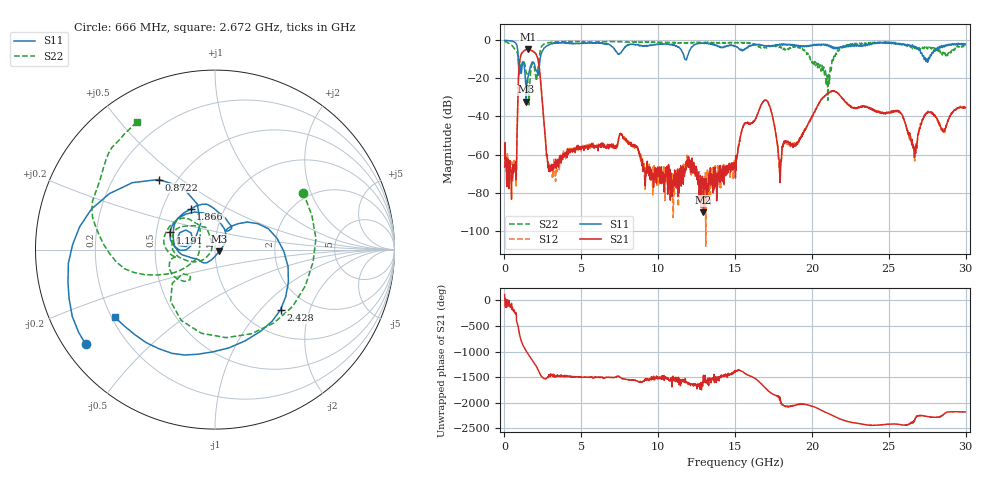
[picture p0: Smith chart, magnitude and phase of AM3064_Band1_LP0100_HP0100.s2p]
# Hz S DB R 50.0
!freq dBS11 angS11 dBS21 angS21 dBS12 angS12 dBS22 angS22
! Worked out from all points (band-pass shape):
!   1600 points, 10 MHz to 29.98 GHz, reference 50 ohm
!   highest |S21| = -4.62 dB at 1.528 GHz (marker M1); lowest = -90.3 dB at 12.94 GHz (marker M2)
!   |S21| within 3 dB of the highest: 1.075 GHz to 2.077 GHz (1.003 GHz wide, 63.6 % of centre)
!   lowest |S11| = -32.2 dB at 1.416 GHz (marker M3), VSWR 1.05, Z = 52.3 - j1.08 ohm
!   |S11| at or under -10 dB: 902.1 MHz to 2.314 GHz (1.412 GHz wide, 87.8 % of centre); 11.76 GHz to 11.84 GHz (80.56 MHz wide, 0.683 % of centre); 27.3928 GHz to 27.45994 GHz (67.14 MHz wide, 0.245 % of centre)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
!   |S22| runs from -33.9 to -0.4 dB; largest |S21 - S12| = 0.0091
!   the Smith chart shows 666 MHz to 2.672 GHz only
!   S11 on the Smith chart (normalised r, x): 666 MHz: 0.06, -0.33; 872.2 MHz: 0.40, +0.42; 1.191 GHz: 0.59, +0.12; 1.866 GHz: 0.69, +0.34; 2.428 GHz: 1.46, -1.30; 2.672 GHz: 0.21, -0.29
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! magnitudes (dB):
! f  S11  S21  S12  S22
! 10 MHz  -0.1  -66.6  -54.9  -0.4
! 666 MHz  -1.0  -66.0  -65.1  -4.6
! 872.2 MHz  -6.0  -30.9  -30.8  -8.4
! 1.191 GHz  -11.4  -6.2  -6.1  -10.8
! 1.416 GHz  -32.2  -4.8  -4.7  -16.8
! 1.528 GHz  -19.5  -4.6  -4.6  -22.1
! 1.866 GHz  -11.6  -5.8  -5.9  -12.1
! 2.428 GHz  -6.1  -29.0  -28.9  -3.0
! 2.672 GHz  -3.4  -53.4  -52.2  -1.6
! 3.028 GHz  -1.8  -67.1  -67.2  -1.0
! 5.015 GHz  -1.4  -56.2  -56.5  -0.7
! 7.639 GHz  -5.6  -49.9  -49.9  -0.7
! 10 GHz  -2.0  -68.6  -69.8  -1.0
! 12.94 GHz  -1.5  -90.3  -75.5  -1.1
! 15 GHz  -3.0  -66.0  -63.4  -1.4
! 16.9 GHz  -2.9  -31.5  -31.5  -3.8
! 17.93 GHz  -2.1  -74.8  -69.3  -3.1
! 19.99 GHz  -2.9  -40.4  -40.2  -11.1
! 25 GHz  -1.0  -37.8  -37.9  -1.2
! 26.68 GHz  -3.1  -59.6  -63.4  -4.2
! 27.45 GHz  -10.3  -38.2  -38.2  -3.6
! 29.98 GHz  -1.9  -35.5  -34.9  -2.9
